ORGANIZATION_BLOCK MAIN:OB1
TITLE=

BEGIN
NETWORK 1
LD Q0.0
A I0.0
O I0.2
A I0.1
AN Q0.1
= Q0.0

NETWORK 2
LD Q0.1
A I0.4
O I0.3
A I0.1
AN Q0.0
= Q0.1

NETWORK 3
LDN Q0.0
AN Q0.1
= Q0.2

NETWORK 4
LD Q0.0
= Q0.3

NETWORK 5
LD Q0.1
= Q0.4

END_ORGANIZATION_BLOCK

